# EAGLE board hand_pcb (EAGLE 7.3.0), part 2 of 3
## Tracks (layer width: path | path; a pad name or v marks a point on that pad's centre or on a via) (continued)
+5V1  (via drill 0.38, 0.39) (continued)
  pour Bottom (isolate 1.016, rank 2): 31.83,93.92 28.32,93.92 27.14,95.07 24.89,97.18 21.18,97.37 18.43,97.42 16.9,97.05 15.72,96.37 13.79,96.62 12.7,97.28 12.74,98.35 13.34,99.09 14.61,99.44 16.41,99.92 18.17,100.56 19.63,101.24 21.48,102.48 22.85,103.77 23.95,105.22 24.83,106.68 25.04,107.37 26.12,113.53 26.47,115.62 26.5,118.2 26.35,119.42 26.21,120.65 25.64,122.83 25.12,124.12 24.78,125.13 24.64,126.11 24.49,128.27 48.49,128.23 50.2,127.74 50.16,125.12 47.47,123.44 43.88,122.17 44.34,115.27 35.92,114.48 33.86,111.98 36.14,106.78 39.55,102.27 42.93,97.64 48.7,97.09 49.76,85.5 34.99,87.38
+5V2  (via drill 0.38, 0.39)
  Top 0.254: THMB2.15 111.18,51.43 110.49,52.12 110.49,55.24 109.67,56.07 107.34,56.07 v105.93,57.48 | PKYRNG2.15 119.56,21.16 119.25,20.85 112.03,20.85 111.76,21.12 111.76,25.86 112.52,26.62 C44.1 112.52,26.4 | 116.99,58.28 C47.1 116.6,59.2 v115.44,60.36 | 115.33,55.67 115.06,55.65 | INDMID2.15 81.54,21.43 80.2,22.77 80.48,26.57 82.16,28.14 82.16,29.65 82.58,30.07 85.8,30.07 87.55,28.32
  Top 0.381: 115.06,55.65 115.06,54.99 THMB2.10 | PKYRNG2.10 115.66,25.58 115.39,25.77 | C44.1 | INDMID2.10 86.06,25.43 86.26,25.45 | 87.52,27.5 87.73,27.72
  Top 0.762: 115.75,56.13 115.33,55.67 | 115.39,25.77 114.68,26.09 | 86.26,25.45 86.47,26.06
  Top 1.016: v133.32,55.52 134.73,55.52 C55.1
  Top 1.27: C42.2 C44.1 | C39.2 87.73,27.72 C41.1 | C47.1 117.39,58.28 C45.2 | 116.99,58.28 116.99,56.79 116.33,56.13 115.75,56.13 | 114.68,26.09 113.81,26.62 C44.1 | 86.47,26.06 87.35,27.09 87.52,27.5
  Top 1.524: C42.2 111.49,27.95 110.98,28.45 110.98,31.17 v111.01,31.19 | v89.98,31.08 88.35,31.08 87.55,29.59 87.55,28.32 87.55,27.89 87.73,27.72
  Top 1.905: 122.02,59.83 121.58,60.29 118.14,60.29 117.39,59.91 117.39,58.28
  Top 2.794: v122.03,58.78 122.02,58.55 122.02,59.83
  Bottom 0.254: v105.93,57.48 105.93,57.45 107.3,56.08 111.16,56.08 v115.44,60.36
  Bottom 1.016: v123.14,57.99 126.18,54.95 U$33.1 132.75,54.95 v133.32,55.52
  Bottom 1.524: 112.14,56.82 111.72,56.4 111.27,56.4 111.12,56.26 110.92,56.26 110.73,56.07 110.43,56.07 110.21,55.85 109.58,55.85 109.03,55.31 108.56,55.31
  Bottom 1.905: 113.53,57.2 113.14,56.82 112.14,56.82
  Bottom 2.794: v111.01,31.19 111.01,32.87 109.97,33.91 | 109.97,33.91 106.46,33.91 106.01,33.45 102.49,33.45 | 102.49,33.45 100.71,33.45 100.03,32.77 96.88,32.77 93.7,31.37 90.96,31.37 v89.98,31.08 | 109.97,33.91 110.01,33.95 | 103.34,40.88 103.34,50.98 | 103.34,50.98 103.34,51.13 | v122.03,58.78 113.51,58.76 113.53,58.75 113.53,57.2 | 108.56,55.31 104.23,50.98 103.34,50.98 | 103.85,40.37 102.49,39.01 102.49,33.45
  Bottom 3.81: U$28.3 106.01,28.65 106.01,33.45
  other vias: 104.85,31.24 107.2,30.19 89.26,30.04 107.24,32.13 111.05,32.58 91.35,30.73 90.98,32.28 88.38,31.34 120.68,59.65 121.31,57.77 123.19,59.35 122.07,60.12 118.66,59.88 117.16,59.92
  pour Top (isolate 0.406): 115.89,25.54 113.96,25.54 113.35,26.15 110.81,26.15 106.27,26.58 104.13,28.26 104.23,32.88 112.31,33.16 112.37,30.8 111.84,30.63 111.84,28.85 112.04,28.65 113.74,28.65 115.62,26.77 115.62,25.86 115.91,25.57
  pour Top (isolate 0.406): 85.98,24.97 85.98,26.64 86.35,27.01 86.35,30.57 88.07,32.03 91.52,32.92 92.11,32.5 92.48,30.91 91.87,30.12 90.61,29.1 88.75,28.96 88.75,26.39 87.85,25.49 86.6,25.49 86.08,24.97
  pour Top (isolate 0.406): 115.02,55.23 115.02,56.52 116,57.49 116,59.08 115.53,59.55 114.97,59.55 114.67,59.86 114.67,60.96 115.23,61.52 122.99,61.52 124.09,60.41 124.09,58.66 122.9,57.47 121.39,57.47 120.73,58.13 120.73,58.93 119.98,59.68 118.99,59.68 118.52,59.21 118.52,56.88 117.21,55.58 116.07,55.58 115.75,55.26 115.07,55.26 115.06,55.24
  pour Bottom (isolate 1.016, rank 2): 106.68,26.76 103.17,26.76 101.99,27.91 99.75,30.02 96.04,30.21 93.28,30.26 91.76,29.9 90.58,29.21 88.65,29.46 87.55,30.12 87.59,31.19 88.19,31.93 89.46,32.28 91.26,32.77 93.03,33.4 94.49,34.09 96.33,35.32 97.7,36.61 98.81,38.06 99.68,39.52 99.9,40.21 100.98,46.37 101.32,48.46 101.36,51.04 101.21,52.26 101.07,53.49 100.5,55.68 99.97,56.96 99.63,57.98 99.49,58.95 99.34,61.11 123.34,61.07 125.06,60.58 125.02,57.96 122.33,56.29 118.73,55.02 119.19,48.11 110.77,47.32 108.71,44.82 111,39.62 114.4,35.12 117.78,30.48 123.56,29.93 124.61,18.34 109.84,20.22
+5V3  (via drill 0.38, 0.39)
  Top 0.254: THMB3.15 110.41,82.05 111.1,81.36 111.1,78.23 111.92,77.41 114.25,77.41 v115.66,76 | PKYRNG3.15 102.03,112.32 102.34,112.62 109.56,112.62 109.83,112.36 109.83,107.62 109.07,106.86 C63.1 109.07,107.07 | 104.6,75.2 C66.1 104.99,74.27 v106.15,73.11 | 106.25,77.81 106.53,77.83 | INDMID3.15 140.05,112.05 141.39,110.71 141.11,106.91 139.43,105.33 139.43,103.82 139.01,103.4 135.79,103.4 134.04,105.16
  Top 0.381: 106.53,77.83 106.53,78.49 THMB3.10 | PKYRNG3.10 105.93,107.9 106.2,107.71 | C63.1 | INDMID3.10 135.53,108.05 135.33,108.03 | 134.07,105.98 133.86,105.76
  Top 0.762: 105.84,77.34 106.25,77.81 | 106.2,107.71 106.91,107.39 | 135.33,108.03 135.12,107.42
  Top 1.016: v88.27,77.95 86.86,77.95 C74.1
  Top 1.27: C61.2 C63.1 | C58.2 133.86,105.76 C60.1 | C66.1 104.2,75.2 C64.2 | 104.6,75.2 104.6,76.68 105.26,77.34 105.84,77.34 | 106.91,107.39 107.78,106.86 C63.1 | 135.12,107.42 134.24,106.39 134.07,105.98
  Top 1.524: C61.2 110.1,105.53 110.6,105.03 110.6,102.31 v110.58,102.29 | v131.61,102.4 133.24,102.4 134.04,103.89 134.04,105.16 134.04,105.58 133.86,105.76
  Top 1.905: 99.57,73.65 100.01,73.19 103.45,73.19 104.2,73.57 104.2,75.2
  Top 2.794: v99.56,74.7 99.57,74.93 99.57,73.65
  Bottom 0.254: v115.66,76 115.66,76.02 114.29,77.39 110.43,77.39 v106.15,73.11
  Bottom 1.016: v98.45,75.49 95.41,78.53 U$45.1 88.84,78.53 v88.27,77.95
  Bottom 1.524: 109.45,76.66 109.87,77.08 110.33,77.08 110.47,77.22 110.67,77.22 110.86,77.41 111.16,77.41 111.38,77.62 112.01,77.62 112.56,78.17 113.03,78.17
  Bottom 1.905: 108.06,76.28 108.44,76.66 109.45,76.66
  Bottom 2.794: v110.58,102.29 110.58,100.61 111.62,99.57 | 111.62,99.57 115.13,99.57 115.58,100.03 119.1,100.03 | 119.1,100.03 120.88,100.03 121.56,100.71 124.71,100.71 127.89,102.11 130.63,102.11 v131.61,102.4 | 111.62,99.57 111.58,99.53 | 118.25,92.6 118.25,82.5 | 118.25,82.5 118.25,82.35 | v99.56,74.7 108.08,74.71 108.06,74.73 108.06,76.28 | 113.03,78.17 117.36,82.5 118.25,82.5 | 117.74,93.1 119.1,94.46 119.1,100.03
  Bottom 3.81: U$40.3 115.58,104.83 115.58,100.03
  other vias: 116.74,102.23 114.39,103.29 132.33,103.44 114.35,101.35 110.54,100.9 130.24,102.74 130.61,101.19 133.21,102.13 100.91,73.83 100.28,75.7 98.4,74.13 99.52,73.36 102.93,73.6 104.43,73.56
  pour Top (isolate 0.406): 105.7,107.94 107.63,107.94 108.24,107.33 110.78,107.33 115.32,106.9 117.46,105.22 117.36,100.6 109.28,100.32 109.22,102.68 109.75,102.84 109.75,104.62 109.55,104.83 107.85,104.83 105.97,106.71 105.97,107.62 105.68,107.91
  pour Top (isolate 0.406): 135.61,108.51 135.61,106.83 135.24,106.46 135.24,102.91 133.52,101.45 130.07,100.56 129.48,100.98 129.11,102.57 129.72,103.35 130.98,104.38 132.84,104.52 132.84,107.09 133.74,107.99 134.99,107.99 135.51,108.51
  pour Top (isolate 0.406): 106.57,78.24 106.57,76.96 105.59,75.98 105.59,74.4 106.06,73.93 106.62,73.93 106.92,73.62 106.92,72.52 106.36,71.96 98.6,71.96 97.5,73.06 97.5,74.82 98.69,76.01 100.2,76.01 100.86,75.35 100.86,74.55 101.61,73.8 102.6,73.8 103.07,74.27 103.07,76.59 104.38,77.9 105.52,77.9 105.84,78.22 106.51,78.22 106.53,78.23
  pour Bottom (isolate 1.016, rank 2): 114.91,106.72 118.41,106.72 119.6,105.56 121.84,103.45 125.55,103.26 128.31,103.21 129.83,103.58 131.01,104.27 132.94,104.01 134.04,103.35 134,102.29 133.4,101.55 132.13,101.19 130.33,100.71 128.56,100.08 127.1,99.39 125.26,98.16 123.89,96.86 122.78,95.42 121.91,93.95 121.69,93.27 120.61,87.11 120.27,85.01 120.23,82.44 120.38,81.22 120.52,79.98 121.09,77.8 121.62,76.52 121.96,75.5 122.1,74.52 122.25,72.36 98.25,72.4 96.53,72.9 96.57,75.51 99.26,77.19 102.86,78.46 102.4,85.37 110.82,86.16 112.88,88.66 110.59,93.85 107.19,98.36 103.81,103 98.03,103.54 96.98,115.14 111.75,113.26
EN1
  Top 0.254: U$1.4 40.5,43.47 41.43,44.4 41.43,48.28 38.48,51.23 37.24,51.23 U$5.1
EN2
  Top 0.254: U$1.5 40.61,42.82 41.88,44.09 41.88,48.49 U$5.2
EN3
  Top 0.254: U$7.1 48.28,41.96 47.42,42.82 U$1.12
EN4
  Top 0.254: U$7.2 49.99,40.92 48.28,40.92 47.03,42.17 U$1.11
EN5  (via drill 0.38)
  Top 0.254: U$1.10 43.67,41.52 42.8,42.39 42.8,45.97 v43.08,46.25
  Bottom 0.254: v43.08,46.25 45.06,46.25 51.66,52.86 U$6.1
EN6  (via drill 0.38)
  Top 0.254: U$1.9 43.56,40.87 42.34,42.09 42.34,46.97 v42.62,47.24
  Bottom 0.254: v42.62,47.24 45.29,47.24 50.44,52.4 50.44,54.86 51.61,56.03 U$6.2
EN7
  Top 0.254: U$13.4 31.25,90.16 30.33,89.23 30.33,85.34 33.27,82.4 34.52,82.4 U$17.1
EN8
  Top 0.254: U$13.5 31.14,90.81 29.87,89.53 29.87,85.14 U$17.2
EN9  (via drill 0.38)
  Top 0.254: U$13.9 28.2,92.76 29.41,91.54 29.41,86.67 v29.13,86.39
  Bottom 0.254: v29.13,86.39 26.47,86.39 21.31,81.23 21.31,78.77 20.14,77.6 U$19.2
EN10
  Top 0.254: U$18.1 23.47,91.67 24.33,90.81 U$13.12
EN11
  Top 0.254: U$18.2 21.77,92.71 23.47,92.71 24.72,91.46 U$13.11
EN12  (via drill 0.38)
  Top 0.254: U$13.10 28.09,92.11 28.96,91.24 28.96,87.66 v28.68,87.38
  Bottom 0.254: v28.68,87.38 26.7,87.38 20.09,80.77 U$19.1
EN13
  Top 0.254: U$25.4 106.11,23 105.18,22.07 105.18,18.19 108.13,15.24 109.37,15.24 U$29.1
EN14
  Top 0.254: U$25.5 106,23.65 104.72,22.38 104.72,17.98 U$29.2
EN15  (via drill 0.38)
  Top 0.254: U$25.9 103.05,25.6 104.27,24.38 104.27,19.51 v103.99,19.23
  Bottom 0.254: v103.99,19.23 101.32,19.23 96.16,14.07 96.16,11.61 95,10.44 U$31.2
EN16
  Top 0.254: U$30.1 98.32,24.51 99.19,23.65 U$25.12
EN17
  Top 0.254: U$30.2 96.62,25.55 98.32,25.55 99.58,24.3 U$25.11
EN18  (via drill 0.38)
  Top 0.254: U$25.10 102.94,24.95 103.81,24.08 103.81,20.5 v103.53,20.22
  Bottom 0.254: v103.53,20.22 101.55,20.22 94.94,13.61 U$31.1
EN19
  Top 0.254: U$37.4 115.48,110.48 116.41,111.4 116.41,115.29 113.46,118.24 112.22,118.24 U$41.1
EN20
  Top 0.254: U$37.5 115.59,109.83 116.86,111.1 116.86,115.49 U$41.2
EN21  (via drill 0.38)
  Top 0.254: U$37.9 118.54,107.88 117.32,109.09 117.32,113.97 v117.6,114.25
  Bottom 0.254: v117.6,114.25 120.27,114.25 125.42,119.41 125.42,121.87 126.59,123.04 U$43.2
EN22
  Top 0.254: U$42.1 123.27,108.97 122.41,109.83 U$37.12
EN23
  Top 0.254: U$42.2 124.97,107.92 123.27,107.92 122.01,109.18 U$37.11
EN24  (via drill 0.38)
  Top 0.254: U$37.10 118.65,108.53 117.78,109.4 117.78,112.98 v118.06,113.26
  Bottom 0.254: v118.06,113.26 120.04,113.26 126.64,119.86 U$43.1
GND  (via drill 0.3, 0.38, 0.39, 1.27)
  Top 0.254: THUMB_A.6 40.18,17.32 40.18,17.78 v40.79,18.39 | v41.83,30.5 41.56,29.7 THUMB_B.6 | BOOTLOADER.2 9.55,20.18 10.46,19.27 10.46,18.39 v10.71,18.15 12.56,18.96 C15.2 | 9.55,22.81 9.88,23.14 BOOTLOADER.PPAD | C15.2 13.42,19.61 | 29.64,41.55 PKYRNG.11 29.67,41.55 30.2,41.53 | PKYRNG.PPAD 27.73,41.22 28.07,41.55 26.94,41.55 v26.87,41.72 | HAND_MICRO.4 24.13,31.62 C14.2 24.38,32.56 v24.38,33.58 | HAND_MICRO.47 25.13,15.78 C16.2 25.4,15.22 v26.06,14.26 | INDMID.PPAD 60.88,44.73 v60.38,45.23 | HAND_MICRO.31 14.58,19.97 14.19,19.57 C15.2 | C15.2 | v47.16,38.08 47.13,38.1 44.32,38.1 41.55,40.87 U$1.8 37.74,40.87 37.06,41.55 C19.2
  Top 0.381: C3.2 61.2,38.91 | C2.2 61.79,37.4 61.37,37.82 C3.2 | PKYRNG.11 31.52,41.54 v32.79,44.01 32.35,41.9 33.45,41.53 C6.2 C5.2 | THMB.PPAD 31.88,14.82 v31.38,15.21 | v33.16,5.64 33.16,6.65 C8.2 33.03,6.87 C9.2 32.2,8.69 THMB.11 | INDMID.11 61.2,41.08 v61.73,40.55 61.35,40.17 C3.2 | INDEX.6 54.42,51.92 v54.41,51.93 | v41.17,52.41 41.66,50.95 42.4,50.86 MIDDLE.6 | RING.6 v25.52,49.76 v25.51,49.76 | v12.45,43.67 12.53,43.76 PINKY.6 13.46,43.72 13.46,41.2 13.42,41.16 13.42,40.4 16.03,37.79 U$3.1 | v5.94,38.28 6.19,38.03 USB.5 | C13.2 12.47,28.77 12.47,29.65 11.19,30.94 10.06,30.94 | 10.06,30.94 v12.12,30.71 | GND.P$1 10.06,30.94 | BOOTLOADER.PPAD 9.28,23.72 v9.28,24.31 v10.46,24.31 v10.46,23.13 v9.27,23.13
  Top 1.016: C17.2 12.08,8.7 v12.5,9.25 11.04,8.7 C18.2
  Route15 0.254: v41.83,30.5 42.34,30.76 44.76,30.76 | v26.87,40.72 26.89,40.73 27.84,40.73 27.85,40.74 27.85,40.84 | v24.38,33.58 25.45,32.51 v29.81,32.51 | v10.71,18.15 10.46,18.39 v10.46,23.13 | U$7.G 50.6,47.24 52.02,47.24 55.27,43.99 55.37,43.99
  Route15 0.381: v32.79,44.01 29.81,39.83 29.81,38.47 | v33.16,5.64 31.38,7.24 v31.38,15.21 | v61.73,40.55 61.73,42.09 60.54,43.28 60.54,45.06 v60.38,45.23 | v54.41,51.93 42.24,51.93 v41.17,52.41 40.07,49.76 v25.51,49.76 | v25.51,49.76 19.43,43.67 v12.45,43.67 12.45,42.99 9.51,39.8 v5.94,38.28 6.48,37.24 7.79,34.59 8.55,33.05 v12.12,30.71 | v25.51,49.76 25.54,49.73 25.54,45.5 26.87,44.17 v26.87,41.72 | v40.79,18.39 41.11,18.71 43.16,18.71
  Route15 0.762: v9.27,23.13 9.3,23.14 10.11,23.95 10.11,24.3 6.69,27.71 6.69,33.49 7.79,34.59
  Route15 1.524: v26.87,41.72 26.86,41.59 27.36,41.1
  Route15 2.794: 44.76,32.11 44.76,30.76 44.76,25.01 43.16,23.41 43.16,18.71 43.16,14.78 43.07,14.87 33.47,14.87 33.12,15.21 v31.38,15.21 | 44.76,32.11 50.87,38.22 53.3,40.4 53.3,41.92 55.37,43.99 55.75,44.37 60.54,44.37 INDMID.PPAD 60.88,44.73 v60.38,45.23 | 44.76,32.11 44.08,32.78 40.4,32.47 40.13,32.21 37.6,32.23 36.94,31.57 33.19,31.57 32.24,32.51 v29.81,32.51 29.81,38.47 29.81,38.65 27.36,41.1
  Route15 3.81: v48.35,38.7 50.87,38.66 50.87,38.22
  Bottom 0.254: v26.06,14.26 27.75,14.41 R5.1 | 35.69,19.79 39.4,19.79 v40.79,18.39 | R15.2 32.89,23.67 33.25,23.42 35.2,23.42 35.72,23.94 R14.2 35.72,26.14 R16.2 40.09,30.5 v41.83,30.5
  Bottom 1.016: U$9.2 U$9.TAB 9.09,11.79 10.08,12.78 10.03,17.48 v10.71,18.15
  Bottom 1.27: v31.38,15.21 31.77,13.79 32.26,13.31 | U$10.G 38.12,45.24 40.08,43.28 43.92,43.28 47.52,39.67
  Bottom 1.524: R9.1 R8.1 28.78,33.54 v29.81,32.51 | R7.1 61.61,43.28 | 61.61,43.28 R6.1 | R5.1 28.85,13.31 32.26,13.31 R4.1 34.95,13.34 | v60.38,45.23 60.35,44.54 61.61,43.28
  Bottom 3.81: U$2.1 43.87,42.76 43.87,42.72 v48.35,38.7
  other vias: 49.7,38.68 48.69,37.49 48.97,40.01 47.41,39.7 60.38,44.21 61.38,44.21 61.38,45.22 32.38,14.21 32.38,15.21 31.38,14.21 27.88,41.72 27.88,40.72 29.13,33.4 29.18,36.5 10.03,15.54 10.03,13.21 65.53,48.44 29.62,35.05 7.04,27.74 42.85,7.16
  pour Route15 (isolate 0.508): 4.58,49.38 6.54,8.14 9.13,5.23 47.61,5.17 47.04,8.65 45.47,13.96 45.59,18.88 46.72,26.29 49.31,30.28 52.29,32.42 56.39,33.57 62.97,35.59 66.56,36.6 67.83,62.98 54.05,63.61 53.73,58.36 23.22,56.78 23.28,50.27
  pour Bottom (isolate 1.016, rank 3): 36.8,49.25 36.8,46.84 37.49,46.15 37.49,41.86 38.61,40.74 43.1,40.74 46.15,37.69 46.15,37.67 47.88,35.94 48.79,35.94 50.6,37.74 50.6,39.78 50.14,40.23 50.14,46.79 47.42,49.5 38.71,49.5
GND1  (via drill 0.3, 0.38, 0.39, 1.27)
  Top 0.254: THUMB_A1.6 31.57,116.31 31.57,115.85 v30.96,115.24 | v29.92,103.12 30.2,103.93 THUMB_B1.6 | BOOTLOADER1.2 62.2,113.45 61.29,114.36 61.29,115.24 v61.05,115.48 59.2,114.67 C34.2 | 62.2,110.82 61.88,110.49 BOOTLOADER1.PPAD | C34.2 58.33,114.02 | 42.12,92.08 PKYRNG1.11 42.09,92.08 41.55,92.1 | PKYRNG1.PPAD 44.03,92.41 43.69,92.08 44.82,92.08 v44.88,91.91 | HAND_MICRO1.4 47.63,102.01 C33.2 47.37,101.07 v47.37,100.05 | HAND_MICRO1.47 46.63,117.85 C35.2 46.35,118.4 v45.7,119.37 | INDMID1.PPAD 10.88,88.89 v11.38,88.41 | HAND_MICRO1.31 57.17,113.66 57.57,114.06 C34.2 | C34.2 | v24.6,95.56 24.62,95.53 27.43,95.53 30.2,92.76 U$13.8 34.01,92.76 34.7,92.08 C38.2
  Top 0.381: C22.2 10.55,94.72 | C21.2 9.97,96.23 10.39,95.81 10.39,94.89 C22.2 | PKYRNG1.11 40.23,92.09 v38.96,89.62 39.41,91.73 38.3,92.1 C25.2 C24.2 | THMB1.PPAD 39.88,118.81 v40.37,118.42 | v38.59,127.99 38.59,126.98 C27.2 38.72,126.76 C28.2 39.55,124.94 THMB1.11 | INDMID1.11 10.55,92.55 v10.02,93.08 10.4,93.46 C22.2 | INDEX1.6 17.33,81.71 v17.35,81.7 | v30.58,81.22 30.1,82.68 29.35,82.77 MIDDLE1.6 | RING1.6 v46.24,83.87 | v59.31,89.95 59.22,89.87 PINKY1.6 58.29,89.91 58.29,92.43 58.33,92.47 58.33,93.23 55.73,95.83 U$14.1 | v65.81,95.35 65.57,95.59 USB1.5 | C32.2 59.28,104.86 59.28,103.97 60.57,102.69 61.7,102.69 | 61.7,102.69 v59.64,102.92 | GND1.P$1 61.7,102.69 | BOOTLOADER1.PPAD 62.47,109.91 v62.47,109.32 v61.29,109.32 v61.29,110.5 v62.48,110.5
  Top 1.016: C36.2 59.68,124.93 v59.26,124.38 60.72,124.93 C37.2
  Route15 0.254: v29.92,103.12 29.41,102.87 27,102.87 | v44.88,92.91 v44.87,92.9 43.92,92.9 43.9,92.89 43.9,92.79 | v47.37,100.05 46.3,101.12 v41.95,101.12 | v61.05,115.48 61.29,115.24 v61.29,110.5 | U$18.G 21.16,86.39 19.74,86.39 16.48,89.64 16.38,89.64
  Route15 0.381: v38.96,89.62 41.95,93.8 41.95,95.16 | v38.59,127.99 40.37,126.39 v40.37,118.42 | v10.02,93.08 10.02,91.54 11.21,90.35 11.21,88.57 v11.38,88.41 | v17.35,81.7 29.52,81.7 v30.58,81.22 31.69,83.87 v46.24,83.87 | v46.24,83.87 52.32,89.95 v59.31,89.95 59.31,90.64 62.24,93.83 v65.81,95.35 65.28,96.39 63.97,99.04 63.21,100.58 v59.64,102.92 | v46.24,83.87 46.22,83.9 46.22,88.12 44.88,89.46 v44.88,91.91 | v30.96,115.24 30.64,114.92 28.6,114.92
  Route15 0.762: v62.48,110.5 62.46,110.49 61.65,109.68 61.65,109.33 65.06,105.92 65.06,100.14 63.97,99.04
  Route15 1.524: v44.88,91.91 44.9,92.04 44.4,92.53
  Route15 2.794: 27,101.52 27,102.87 27,108.62 28.6,110.22 28.6,114.92 28.6,118.85 28.69,118.76 38.29,118.76 38.63,118.42 v40.37,118.42 | 27,101.52 20.89,95.41 18.45,93.23 18.45,91.71 16.38,89.64 16,89.26 11.22,89.26 INDMID1.PPAD 10.88,88.89 v11.38,88.41 | 27,101.52 27.67,100.85 31.36,101.16 31.62,101.42 34.15,101.4 34.81,102.06 38.57,102.06 39.51,101.12 v41.95,101.12 41.95,95.16 41.95,94.98 44.4,92.53
  Route15 3.81: v23.41,94.93 20.89,94.96 20.89,95.41
  Bottom 0.254: v45.7,119.37 44.01,119.22 R21.1 | 36.07,113.84 32.36,113.84 v30.96,115.24 | R31.2 38.86,109.96 38.51,110.21 36.55,110.21 36.03,109.69 R30.2 36.03,107.49 R32.2 31.66,103.12 v29.92,103.12
  Bottom 1.016: U$21.2 U$21.TAB 62.66,121.84 61.67,120.85 61.72,116.15 v61.05,115.48
  Bottom 1.27: v40.37,118.42 39.98,119.84 39.5,120.32 | U$22.G 33.63,88.39 31.67,90.35 27.84,90.35 24.23,93.95
  Bottom 1.524: R25.1 R24.1 42.98,100.09 v41.95,101.12 | R23.1 10.15,90.35 | 10.15,90.35 R22.1 | R21.1 42.9,120.32 39.5,120.32 R20.1 36.8,120.29 | v11.38,88.41 11.4,89.09 10.15,90.35
  Bottom 3.81: U$16.1 27.89,90.87 27.89,90.91 v23.41,94.93
  other vias: 22.06,94.95 23.06,96.14 22.78,93.62 24.35,93.93 11.38,89.42 10.38,89.42 10.38,88.4 39.37,119.42 39.37,118.41 40.37,119.42 43.88,91.91 43.88,92.91 42.62,100.23 42.57,97.13 61.72,118.08 61.72,120.42 6.22,85.19 42.14,98.58 64.72,105.89 28.91,126.47
  pour Route15 (isolate 0.508): 67.17,84.25 65.21,125.49 62.62,128.4 24.14,128.46 24.71,124.98 26.29,119.67 26.16,114.74 25.03,107.34 22.44,103.35 19.47,101.21 15.37,100.06 8.79,98.04 5.19,97.03 3.92,70.65 17.7,70.02 18.02,75.27 48.54,76.85 48.48,83.36
  pour Bottom (isolate 1.016, rank 3): 34.95,84.38 34.95,86.79 34.26,87.48 34.26,91.77 33.15,92.89 28.65,92.89 25.6,95.94 25.6,95.96 23.88,97.69 22.96,97.69 21.16,95.89 21.16,93.85 21.62,93.4 21.62,86.84 24.33,84.12 33.05,84.12
GND2  (via drill 0.3, 0.38, 0.39, 1.27)
  Top 0.254: THUMB_A2.6 106.43,49.15 106.43,48.69 v105.82,48.08 | v104.78,35.97 105.05,36.78 THUMB_B2.6 | BOOTLOADER2.2 137.06,46.29 136.14,47.21 136.14,48.08 v135.9,48.32 134.05,47.51 C53.2 | 137.06,43.66 136.73,43.34 BOOTLOADER2.PPAD | C53.2 133.19,46.86 | 116.97,24.92 PKYRNG2.11 116.94,24.92 116.41,24.94 | PKYRNG2.PPAD 118.88,25.25 118.54,24.92 119.67,24.92 v119.74,24.75 | HAND_MICRO2.4 122.48,34.85 C52.2 122.22,33.91 v122.22,32.89 | HAND_MICRO2.47 121.48,50.69 C54.2 121.21,51.25 v120.55,52.21 | INDMID2.PPAD 85.73,21.74 v86.23,21.25 | HAND_MICRO2.31 132.03,46.51 132.42,46.9 C53.2 | C53.2 | v99.45,28.4 99.48,28.37 102.29,28.37 105.06,25.6 U$25.8 108.87,25.6 109.55,24.92 C57.2
  Top 0.381: C41.2 85.41,27.57 | C40.2 84.82,29.07 85.24,28.65 C41.2 | PKYRNG2.11 115.09,24.93 v113.82,22.47 114.26,24.57 113.16,24.94 C44.2 C43.2 | THMB2.PPAD 114.73,51.65 v115.23,51.26 | v113.45,60.83 113.45,59.82 C46.2 113.57,59.6 C47.2 114.41,57.78 THMB2.11 | INDMID2.11 85.41,25.39 v84.87,25.92 85.25,26.3 C41.2 | INDEX2.6 92.19,14.55 v92.2,14.54 | v105.44,14.06 104.95,15.52 104.21,15.61 MIDDLE2.6 | RING2.6 v121.09,16.71 | v134.16,22.8 134.08,22.71 PINKY2.6 133.15,22.75 133.15,25.27 133.19,25.31 133.19,26.07 130.58,28.68 U$26.1 | v140.66,28.19 140.42,28.44 USB2.5 | C51.2 134.14,37.7 134.14,36.82 135.42,35.53 136.55,35.53 | 136.55,35.53 v134.49,35.76 | GND2.P$1 136.55,35.53 | BOOTLOADER2.PPAD 137.32,42.76 v137.32,42.16 v136.14,42.16 v136.14,43.34 v137.34,43.34
  Top 1.016: C55.2 134.53,57.77 v134.11,57.23 135.57,57.77 C56.2
  Route15 0.254: v104.78,35.97 104.27,35.71 101.85,35.71 | v119.74,25.76 119.72,25.74 118.77,25.74 118.76,25.73 118.76,25.63 | v122.22,32.89 121.16,33.96 v116.8,33.96 | v135.9,48.32 136.14,48.08 v136.14,43.34 | U$30.G 96.01,19.23 94.59,19.23 91.34,22.48 91.24,22.48
  Route15 0.381: v113.82,22.47 116.8,26.64 116.8,28 | v113.45,60.83 115.23,59.23 v115.23,51.26 | v84.87,25.92 84.87,24.38 86.07,23.19 86.07,21.41 v86.23,21.25 | v92.2,14.54 104.37,14.54 v105.44,14.06 106.54,16.71 v121.09,16.71 | v121.09,16.71 127.18,22.8 v134.16,22.8 134.16,23.48 137.1,26.67 v140.66,28.19 140.13,29.23 138.82,31.89 138.06,33.43 v134.49,35.76 | v121.09,16.71 121.07,16.74 121.07,20.97 119.74,22.3 v119.74,24.75 | v105.82,48.08 105.5,47.77 103.45,47.77
  Route15 0.762: v137.34,43.34 137.31,43.33 136.5,42.52 136.5,42.18 139.92,38.76 139.92,32.98 138.82,31.89
  Route15 1.524: v119.74,24.75 119.75,24.88 119.25,25.38
  Route15 2.794: 101.85,34.37 101.85,35.71 101.85,41.47 103.45,43.07 103.45,47.77 103.45,51.69 103.54,51.6 113.14,51.6 113.49,51.26 v115.23,51.26 | 101.85,34.37 95.74,28.25 93.31,26.07 93.31,24.55 91.24,22.48 90.86,22.1 86.07,22.1 INDMID2.PPAD 85.73,21.74 v86.23,21.25 | 101.85,34.37 102.53,33.69 106.21,34 106.48,34.27 109,34.24 109.67,34.9 113.42,34.9 114.36,33.96 v116.8,33.96 116.8,28 116.8,27.83 119.25,25.38
  Route15 3.81: v98.26,27.77 95.74,27.81 95.74,28.25
  Bottom 0.254: v120.55,52.21 118.86,52.06 R37.1 | 110.92,46.69 107.21,46.69 v105.82,48.08 | R47.2 113.72,42.8 113.36,43.05 111.4,43.05 110.89,42.53 R46.2 110.89,40.34 R48.2 106.52,35.97 v104.78,35.97
  Bottom 1.016: U$33.2 U$33.TAB 137.51,54.69 136.53,53.7 136.57,48.99 v135.9,48.32
  Bottom 1.27: v115.23,51.26 114.83,52.68 114.35,53.16 | U$34.G 108.48,21.23 106.53,23.19 102.69,23.19 99.08,26.8
  Bottom 1.524: R41.1 R40.1 117.83,32.93 v116.8,33.96 | R39.1 85,23.19 | 85,23.19 R38.1 | R37.1 117.75,53.16 114.35,53.16 R36.1 111.66,53.14 | v86.23,21.25 86.26,21.93 85,23.19
  Bottom 3.81: U$28.1 102.74,23.71 102.74,23.75 v98.26,27.77
  other vias: 96.91,27.79 97.92,28.98 97.64,26.47 99.2,26.77 86.23,22.26 85.23,22.26 85.23,21.25 114.22,52.26 114.22,51.26 115.23,52.26 118.73,24.75 118.73,25.76 117.47,33.07 117.42,29.97 136.58,50.93 136.58,53.26 81.08,18.03 116.99,31.42 139.57,38.73 103.76,59.31
  pour Route15 (isolate 0.508): 142.02,17.09 140.07,58.33 137.48,61.24 99,61.3 99.57,57.82 101.14,52.51 101.02,47.59 99.89,40.18 97.29,36.2 94.32,34.05 90.22,32.91 83.64,30.89 80.05,29.87 78.78,3.49 92.56,2.86 92.88,8.12 123.39,9.69 123.33,16.21
  pour Bottom (isolate 1.016, rank 3): 109.8,17.22 109.8,19.63 109.12,20.32 109.12,24.61 108,25.73 103.5,25.73 100.46,28.78 100.46,28.8 98.73,30.53 97.82,30.53 96.01,28.73 96.01,26.7 96.47,26.24 96.47,19.68 99.19,16.97 107.9,16.97
GND3  (via drill 0.3, 0.38, 0.39, 1.27)
  Top 0.254: THUMB_A3.6 115.16,84.33 115.16,84.78 v115.77,85.39 | v116.81,97.51 116.54,96.7 THUMB_B3.6 | BOOTLOADER3.2 84.53,87.18 85.45,86.27 85.45,85.39 v85.69,85.15 87.54,85.97 C72.2 | 84.53,89.81 84.86,90.14 BOOTLOADER3.PPAD | C72.2 88.4,86.61 | PKYRNG3.11 104.65,108.56 105.18,108.53 | PKYRNG3.PPAD 102.71,108.22 103.05,108.56 101.92,108.56 v101.85,108.72 | HAND_MICRO3.4 99.11,98.62 C71.2 99.36,99.57 v99.36,100.58 | HAND_MICRO3.47 100.11,82.78 C73.2 100.38,82.23 v101.04,81.27 | INDMID3.PPAD 135.86,111.74 v135.36,112.23 | HAND_MICRO3.31 89.56,86.97 89.17,86.58 C72.2 | C72.2 | v122.14,105.08 122.11,105.11 119.3,105.11 116.53,107.88 U$37.8 112.72,107.88 112.04,108.56 C76.2
  Top 0.381: C60.2 136.18,105.91 | C59.2 136.77,104.41 136.35,104.83 136.35,105.75 C60.2 | PKYRNG3.11 106.5,108.55 v107.77,111.01 107.33,108.9 108.43,108.53 C63.2 C62.2 | THMB3.PPAD 106.86,81.83 v106.36,82.22 | v108.14,72.64 108.14,73.65 C65.2 108.02,73.87 C66.2 107.18,75.7 THMB3.11 | INDMID3.11 136.18,108.09 v136.72,107.56 136.34,107.18 C60.2 | INDEX3.6 129.4,118.92 v129.39,118.94 | v116.15,119.42 116.64,117.96 117.38,117.87 MIDDLE3.6 | RING3.6 v100.5,116.77 v100.5,116.76 | v87.43,110.68 87.51,110.77 PINKY3.6 88.44,110.73 88.44,108.2 88.41,108.17 88.41,107.4 91.01,104.8 U$38.1 | v80.92,105.28 81.17,105.04 USB3.5 | C70.2 87.45,95.78 87.45,96.66 86.17,97.94 85.04,97.94 | 85.04,97.94 v87.1,97.71 | GND3.P$1 85.04,97.94 | BOOTLOADER3.PPAD 84.26,90.72 v84.26,91.31 v85.45,91.31 v85.45,90.13 v84.25,90.13
  Top 1.016: C74.2 87.06,75.71 v87.48,76.25 86.02,75.7 C75.2
  Route15 0.254: v116.81,97.51 117.32,97.77 119.74,97.77 | v101.85,107.72 101.87,107.73 102.82,107.73 102.83,107.75 102.83,107.85 | v99.36,100.58 100.43,99.52 v104.79,99.52 | v85.69,85.15 85.45,85.39 v85.45,90.13 | U$42.G 125.58,114.25 127,114.25 130.25,111 130.35,111
  Route15 0.381: v107.77,111.01 104.79,106.83 104.79,105.47 | v108.14,72.64 106.36,74.24 v106.36,82.22 | v136.72,107.56 136.72,109.09 135.52,110.29 135.52,112.06 v135.36,112.23 | v129.39,118.94 117.22,118.94 v116.15,119.42 115.05,116.76 v100.5,116.76 | v100.5,116.76 94.41,110.68 v87.43,110.68 87.43,110 84.49,106.81 v80.92,105.28 81.46,104.24 82.77,101.59 83.53,100.05 v87.1,97.71 | v100.5,116.76 100.52,116.74 100.52,112.51 101.85,111.18 v101.85,108.72 | v115.77,85.39 116.09,85.71 118.14,85.71
  Route15 0.762: v84.25,90.13 84.28,90.14 85.09,90.96 85.09,91.3 81.67,94.72 81.67,100.5 82.77,101.59
  Route15 1.524: v101.85,108.72 101.84,108.6 102.34,108.1
  Route15 2.794: 119.74,99.11 119.74,97.77 119.74,92.01 118.14,90.41 118.14,85.71 118.14,81.79 118.05,81.88 108.44,81.88 108.1,82.22 v106.36,82.22 | 119.74,99.11 125.85,105.23 128.28,107.4 128.28,108.93 130.35,111 130.73,111.38 135.52,111.38 INDMID3.PPAD 135.86,111.74 v135.36,112.23 | 119.74,99.11 119.06,99.78 115.38,99.48 115.11,99.21 112.58,99.24 111.92,98.58 108.17,98.58 107.23,99.52 v104.79,99.52 104.79,105.47 104.79,105.65 102.34,108.1
  Route15 3.81: v123.33,105.7 125.85,105.67 125.85,105.23
  Bottom 0.254: v101.04,81.27 102.73,81.42 R53.1 | 110.67,86.79 114.38,86.79 v115.77,85.39 | R63.2 107.87,90.68 108.23,90.42 110.19,90.42 110.7,90.94 R62.2 110.7,93.14 R64.2 115.07,97.51 v116.81,97.51
  Bottom 1.016: U$45.2 U$45.TAB 84.08,78.79 85.06,79.78 85.02,84.48 v85.69,85.15
  Bottom 1.27: v106.36,82.22 106.76,80.8 107.24,80.31 | U$46.G 113.11,112.24 115.06,110.29 118.9,110.29 122.5,106.68
  Bottom 1.524: R57.1 R56.1 103.76,100.55 v104.79,99.52 | R55.1 136.59,110.29 | 136.59,110.29 R54.1 | R53.1 103.83,80.31 107.24,80.31 R52.1 109.93,80.34 | v135.36,112.23 135.33,111.54 136.59,110.29
  Bottom 3.81: U$40.1 118.85,109.77 118.85,109.73 v123.33,105.7
  other vias: 124.68,105.69 123.67,104.5 123.95,107.01 122.39,106.71 135.36,111.21 136.36,111.21 136.36,112.23 107.37,81.22 107.37,82.22 106.36,81.22 102.86,108.72 102.86,107.72 104.11,100.41 104.17,103.5 85.01,82.55 85.01,80.21 140.51,115.44 104.6,102.06 82.02,94.74 117.83,74.17
  pour Route15 (isolate 0.508): 79.57,116.38 81.52,75.15 84.11,72.24 122.59,72.17 122.02,75.65 120.45,80.96 120.57,85.89 121.7,93.29 124.29,97.28 127.27,99.43 131.37,100.57 137.95,102.59 141.54,103.61 142.81,129.98 129.03,130.62 128.71,125.36 98.2,123.79 98.26,117.27
  pour Bottom (isolate 1.016, rank 3): 111.79,116.26 111.79,113.84 112.47,113.16 112.47,108.86 113.59,107.75 118.08,107.75 121.13,104.7 121.13,104.67 122.86,102.95 123.77,102.95 125.58,104.75 125.58,106.78 125.12,107.24 125.12,113.79 122.4,116.51 113.69,116.51
IDX1
  Top 0.254: 63.75,46.02 INDMID.16
  Top 0.635: 63.75,46.02 64.06,46.79 64.01,48.34 62.81,48.92 62.81,50.19 61.38,51.59 INDEX.1
IDX2
  Top 0.254: INDMID.2 61.21,46.99
  Top 0.381: 61.21,46.99 61.21,47.83 61.47,48.67
  Top 0.635: 61.47,48.67 61.47,49.17 60.66,49.94 60.18,50.32 INDEX.2
IDX3
  Top 0.254: 8,87.61 INDMID1.16
  Top 0.635: 8,87.61 7.7,86.84 7.75,85.29 8.94,84.71 8.94,83.44 10.38,82.04 INDEX1.1
IDX4
  Top 0.254: INDMID1.2
  Top 0.381: INDMID1.2 10.54,85.8 10.29,84.96
  Top 0.635: 10.29,84.96 10.29,84.45 11.1,83.69 11.58,83.31 INDEX1.2
IDX5
  Top 0.254: 82.86,20.45 INDMID2.16
  Top 0.635: 82.86,20.45 82.55,19.68 82.6,18.14 83.8,17.55 83.8,16.28 85.23,14.88 INDEX2.1
IDX6
  Top 0.254: INDMID2.2 85.39,19.48
  Top 0.381: 85.39,19.48 85.39,18.64 85.14,17.8
  Top 0.635: 85.14,17.8 85.14,17.3 85.95,16.54 86.43,16.15 INDEX2.2
IDX7
  Top 0.254: 138.74,113.03 INDMID3.16
  Top 0.635: 138.74,113.03 139.04,113.79 138.99,115.34 137.79,115.93 137.79,117.2 136.36,118.59 INDEX3.1
IDX8
  Top 0.254: INDMID3.2 136.19,114
  Top 0.381: 136.19,114 136.19,114.83 136.45,115.67
  Top 0.635: 136.45,115.67 136.45,116.18 135.64,116.94 135.16,117.32 INDEX3.2
IDXENC1  (via drill 0.38)
  Top 0.254: INDEX.5 v56.5,50.44 | HAND_MICRO.58 29.99,23.97 v30.71,24.69
  Route2 0.254: v30.71,24.69 42.04,24.69 54.48,37.13 54.48,46.25 57.15,48.92 57.15,49.8 v56.5,50.44
IDXENC2  (via drill 0.38)
  Top 0.254: INDEX.4 57.78,51.07 v57.78,50.39 | HAND_MICRO.57 26.06,23.47 v25.27,22.68
  Route2 0.254: v25.27,22.68 26.04,23.44 30.63,23.44 31.39,24.21 42.29,24.21 54.94,36.85 54.94,45.95 57.61,48.62 v57.78,50.39
IDXENC3  (via drill 0.38)
  Top 0.254: INDEX1.4 13.98,82.56 v13.97,83.24 | HAND_MICRO1.57 45.7,110.16 v46.48,110.95
  Route2 0.254: v46.48,110.95 45.72,110.19 41.12,110.19 40.36,109.42 29.46,109.42 16.82,96.77 16.82,87.68 14.15,85.01 v13.97,83.24
IDXENC4  (via drill 0.38)
  Top 0.254: INDEX1.5 v15.25,83.19 | HAND_MICRO1.58 41.77,109.66 v41.05,108.94
  Route2 0.254: v41.05,108.94 29.72,108.94 17.27,96.5 17.27,87.38 14.61,84.71 14.61,83.83 v15.25,83.19
IDXENC5  (via drill 0.38)
  Top 0.254: INDEX2.4 88.83,15.4 v88.82,16.08 | HAND_MICRO2.57 120.55,43.01 v121.34,43.79
  Route2 0.254: v121.34,43.79 120.57,43.03 115.98,43.03 115.21,42.27 104.32,42.27 91.67,29.62 91.67,20.52 89,17.86 v88.82,16.08
IDXENC6  (via drill 0.38)
  Top 0.254: INDEX2.5 v90.11,16.03 | HAND_MICRO2.58 116.62,42.51 v115.9,41.78
  Route2 0.254: v115.9,41.78 104.57,41.78 92.13,29.34 92.13,20.22 89.46,17.55 89.46,16.67 v90.11,16.03
IDXENC7  (via drill 0.38)
  Top 0.254: INDEX3.4 132.76,118.08 v132.77,117.4 | HAND_MICRO3.57 101.04,90.47 v100.25,89.69
  Route2 0.254: v100.25,89.69 101.02,90.45 105.61,90.45 106.38,91.21 117.27,91.21 129.92,103.86 129.92,112.95 132.59,115.62 v132.77,117.4
IDXENC8  (via drill 0.38)
  Top 0.254: INDEX3.5 v131.48,117.45 | HAND_MICRO3.58 104.97,90.97 v105.69,91.69
  Route2 0.254: v105.69,91.69 117.02,91.69 129.46,104.14 129.46,113.26 132.13,115.93 132.13,116.8 v131.48,117.45
IDXISEN  (via drill 0.38)
  Top 0.381: INDMID.1 62.08,47.57
  Top 0.635: 62.08,47.57 v62.74,47.47
  Bottom 0.635: v62.74,47.47 63.93,46.28 R6.2
IDXISEN1  (via drill 0.38)
  Top 0.381: INDMID1.1 9.68,86.06
  Top 0.635: 9.68,86.06 v9.02,86.16
  Bottom 0.635: v9.02,86.16 7.82,87.35 R22.2
IDXISEN2  (via drill 0.38)
  Top 0.381: INDMID2.1 84.53,18.9
  Top 0.635: 84.53,18.9 v83.87,19
  Bottom 0.635: v83.87,19 82.68,20.19 R38.2
IDXISEN3  (via drill 0.38)
  Top 0.381: INDMID3.1 137.06,114.58
  Top 0.635: 137.06,114.58 v137.72,114.48
  Bottom 0.635: v137.72,114.48 138.91,113.28 R54.2
IDXPWM1  (via drill 0.38)
  Top 0.254: INDMID.14 64.65,44.39 65.76,43.28 65.44,40.64 v64.87,40.02 | HAND_MICRO.61 28.97,25.47 34.8,31.29 48.49,31.29 55.63,38.43 55.63,40.36 v55.85,40.36
  Route2 0.254: 65.02,40.16 v64.87,40.02 63.45,38.58 57.33,38.58 v55.85,40.36
IDXPWM2  (via drill 0.38)
  Top 0.254: INDMID.13 63.15,42.77 v64.59,41.33 | HAND_MICRO.62 27.67,25.96 28.73,25.96 34.54,31.77 48.28,31.77 55.14,38.63 55.14,40.82 v55.73,41.4
  Route2 0.254: v55.73,41.4 64.54,41.38 v64.59,41.33
IDXPWM3  (via drill 0.38)
  Top 0.254: INDMID1.13 8.6,90.86 v7.16,92.3 | HAND_MICRO1.62 44.08,107.67 43.03,107.67 37.21,101.85 23.47,101.85 16.61,95 16.61,92.81 v16.03,92.23
  Route2 0.254: v16.03,92.23 7.21,92.25 v7.16,92.3
IDXPWM4  (via drill 0.38)
  Top 0.254: INDMID1.14 7.1,89.24 5.99,90.35 6.31,92.99 v6.88,93.61 | HAND_MICRO1.61 42.78,108.16 36.96,102.34 23.27,102.34 16.13,95.2 16.13,93.27 v15.9,93.27
  Route2 0.254: 6.73,93.47 v6.88,93.61 8.31,95.05 14.43,95.05 v15.9,93.27
IDXPWM5  (via drill 0.38)
  Top 0.254: INDMID2.13 83.46,23.71 v82.02,25.15 | HAND_MICRO2.62 118.94,40.51 117.88,40.51 112.06,34.7 98.32,34.7 91.47,27.84 91.47,25.65 v90.88,25.07
  Route2 0.254: v90.88,25.07 82.07,25.09 v82.02,25.15
IDXPWM6  (via drill 0.38)
  Top 0.254: INDMID2.14 81.96,22.08 80.85,23.19 81.17,25.83 v81.74,26.45 | HAND_MICRO2.61 117.64,41.01 111.81,35.18 98.12,35.18 90.98,28.04 90.98,26.11 v90.75,26.11
  Route2 0.254: 81.58,26.31 v81.74,26.45 83.16,27.89 89.28,27.89 v90.75,26.11
IDXPWM7  (via drill 0.38)
  Top 0.254: INDMID3.13 138.13,109.77 v139.57,108.33 | HAND_MICRO3.62 102.65,92.96 103.71,92.96 109.53,98.78 123.27,98.78 130.12,105.64 130.12,107.82 v130.71,108.41
  Route2 0.254: v130.71,108.41 139.52,108.38 v139.57,108.33
IDXPWM8  (via drill 0.38)
  Top 0.254: INDMID3.14 139.63,111.4 140.74,110.29 140.42,107.64 v139.85,107.02 | HAND_MICRO3.61 103.95,92.47 109.78,98.3 123.47,98.3 130.61,105.44 130.61,107.37 v130.84,107.37
  Route2 0.254: 140,107.16 v139.85,107.02 138.43,105.59 132.31,105.59 v130.84,107.37
LED0
  Top 0.254: HAND_MICRO.53 29.01,21.47 30.94,23.39 31.29,23.39 31.9,24 31.9,24.28 32.55,24.93 RED.1
LED1
  Top 0.254: GREEN.1 32.11,26.72 32.11,26.36 31.7,25.96 31.7,25.25 31.45,24.99 31.45,24.31 30.99,23.85 30.61,23.85 28.72,21.97 HAND_MICRO.54
LED2
  Top 0.254: HAND_MICRO.52 29.27,20.97 31.24,22.94 32.33,22.94 33.25,23.85 35.79,23.85 37.31,26.54 37.31,27.48 YELLOW.1
LED3
  Top 0.254: HAND_MICRO1.53 42.74,112.16 40.82,110.24 40.46,110.24 39.85,109.63 39.85,109.35 39.2,108.69 RED1.1
LED4
  Top 0.254: GREEN1.1 39.65,106.91 39.65,107.26 40.06,107.67 40.06,108.38 40.31,108.64 40.31,109.32 40.77,109.78 41.15,109.78 43.03,111.66 HAND_MICRO1.54
LED5
  Top 0.254: HAND_MICRO1.52 42.48,112.66 40.51,110.69 39.42,110.69 38.51,109.78 35.97,109.78 34.44,107.09 34.44,106.16 YELLOW1.1
LED6
  Top 0.254: HAND_MICRO2.53 117.6,45.01 115.67,43.08 115.32,43.08 114.71,42.47 114.71,42.19 114.05,41.54 RED2.1
LED7
  Top 0.254: GREEN2.1 114.5,39.75 114.5,40.11 114.91,40.51 114.91,41.22 115.16,41.48 115.16,42.16 115.62,42.62 116,42.62 117.89,44.51 HAND_MICRO2.54
LED8
  Top 0.254: HAND_MICRO2.52 117.34,45.51 115.37,43.54 114.28,43.54 113.36,42.62 110.82,42.62 109.3,39.93 109.3,39 YELLOW2.1
LED9
  Top 0.254: HAND_MICRO3.53 103.99,88.47 105.92,90.4 106.27,90.4 106.88,91.01 106.88,91.29 107.53,91.94 RED3.1
LED10
  Top 0.254: GREEN3.1 107.09,93.73 107.09,93.37 106.68,92.96 106.68,92.25 106.43,92 106.43,91.31 105.97,90.86 105.59,90.86 103.7,88.97 HAND_MICRO3.54
LED11
  Top 0.254: HAND_MICRO3.52 104.25,87.97 106.22,89.94 107.31,89.94 108.23,90.86 110.77,90.86 112.29,93.55 112.29,94.48 YELLOW3.1
MID1
  Top 0.381: INDMID.5 58.55,45.87
  Top 0.635: 58.55,45.87 57.33,46.05 56.67,46.97 55.02,47.93 52.93,50.01 47.4,50.01 MIDDLE.2
MID2
  Top 0.254: INDMID.3 60.53,46.99
  Top 0.381: 60.53,46.99 60.53,48.41
  Top 0.635: 60.53,48.41 60.17,48.62 59.31,49.1 55.55,49.1 53.57,51.08 MIDDLE.1
MID3
  Top 0.254: INDMID1.3 11.23,86.64
  Top 0.381: 11.23,86.64 11.23,85.22
  Top 0.635: 11.23,85.22 11.58,85.01 12.45,84.53 16.2,84.53 18.19,82.55 MIDDLE1.1
MID4
  Top 0.381: INDMID1.5 13.21,87.76
  Top 0.635: 13.21,87.76 14.43,87.58 15.09,86.67 16.74,85.7 18.82,83.62 24.36,83.62 MIDDLE1.2
MID5
  Top 0.254: INDMID2.3 86.08,19.48
  Top 0.381: 86.08,19.48 86.08,18.06
  Top 0.635: 86.08,18.06 86.44,17.86 87.3,17.37 91.06,17.37 93.04,15.39 MIDDLE2.1
MID6
  Top 0.381: INDMID2.5 88.06,20.6
  Top 0.635: 88.06,20.6 89.28,20.42 89.94,19.51 91.59,18.54 93.67,16.46 99.21,16.46 MIDDLE2.2
MID7
  Top 0.254: INDMID3.3 135.51,114
  Top 0.381: 135.51,114 135.51,115.42
  Top 0.635: 135.51,115.42 135.15,115.62 134.29,116.1 130.53,116.1 128.55,118.08 MIDDLE3.1
MID8
  Top 0.381: INDMID3.5 133.53,112.87
  Top 0.635: 133.53,112.87 132.31,113.06 131.65,113.97 130,114.94 127.91,117.02 122.38,117.02 MIDDLE3.2
MIDENC1  (via drill 0.38, 0.39)
  Top 0.254: v43.64,49.43 43.7,49.65 MIDDLE.5 | v31.22,26.62 30.86,26.62 29.21,24.97 HAND_MICRO.60
  Route2 0.254: v43.64,49.43 44.88,48.18 51.33,48.18 53.57,45.95 53.57,37.69 41.53,25.65 32.18,25.65 v31.22,26.62
MIDENC2  (via drill 0.38, 0.39)
  Top 0.254: MIDDLE.4 44.73,50.72 v44.73,49.58 | v30.96,25.65 30.63,25.65 29.45,24.47 HAND_MICRO.59
  Route2 0.254: v44.73,49.58 45.67,48.64 51.64,48.64 54.03,46.25 54.03,37.41 41.78,25.17 31.45,25.17 v30.96,25.65
MIDENC3  (via drill 0.38, 0.39)
  Top 0.254: MIDDLE1.4 27.03,82.91 v27.03,84.05 | v40.79,107.97 41.12,107.97 42.31,109.16 HAND_MICRO1.59
  Route2 0.254: v27.03,84.05 26.09,84.99 20.12,84.99 17.73,87.38 17.73,96.22 29.97,108.46 40.31,108.46 v40.79,107.97
MIDENC4  (via drill 0.38, 0.39)
  Top 0.254: v28.12,84.2 28.05,83.98 MIDDLE1.5 | v40.54,107.01 40.89,107.01 42.55,108.66 HAND_MICRO1.60
  Route2 0.254: v28.12,84.2 26.87,85.45 20.42,85.45 18.19,87.68 18.19,95.94 30.23,107.97 39.57,107.97 v40.54,107.01
MIDENC5  (via drill 0.38, 0.39)
  Top 0.254: MIDDLE2.4 101.88,15.75 v101.88,16.89 | v115.65,40.82 115.98,40.82 117.16,42.01 HAND_MICRO2.59
  Route2 0.254: v101.88,16.89 100.94,17.83 94.97,17.83 92.58,20.22 92.58,29.06 104.83,41.3 115.16,41.3 v115.65,40.82
MIDENC6  (via drill 0.38, 0.39)
  Top 0.254: v102.97,17.04 102.91,16.83 MIDDLE2.5 | v115.39,39.85 115.75,39.85 117.4,41.51 HAND_MICRO2.60
  Route2 0.254: v102.97,17.04 101.73,18.29 95.28,18.29 93.04,20.52 93.04,28.78 105.08,40.82 114.43,40.82 v115.39,39.85
MIDENC7  (via drill 0.38, 0.39)
  Top 0.254: MIDDLE3.4 119.71,117.72 v119.71,116.59 | v105.94,92.66 105.61,92.66 104.43,91.47 HAND_MICRO3.59
  Route2 0.254: v119.71,116.59 120.65,115.65 126.62,115.65 129.01,113.26 129.01,104.42 116.76,92.18 106.43,92.18 v105.94,92.66
MIDENC8  (via drill 0.38, 0.39)
  Top 0.254: v118.62,116.43 118.68,116.65 MIDDLE3.5 | v106.2,93.62 105.84,93.62 104.19,91.97 HAND_MICRO3.60
  Route2 0.254: v118.62,116.43 119.86,115.19 126.31,115.19 128.55,112.95 128.55,104.7 116.51,92.66 107.16,92.66 v106.2,93.62
MIDISEN  (via drill 0.38)
  Top 0.381: INDMID.4 59.7,47.47
  Top 0.635: 59.7,47.47 v58.8,47.7
  Bottom 0.635: v58.8,47.7 57.84,46.74 R7.2
MIDISEN1  (via drill 0.38)
  Top 0.381: INDMID1.4 12.05,86.16
  Top 0.635: 12.05,86.16 v12.95,85.93
  Bottom 0.635: v12.95,85.93 13.92,86.89 R23.2
MIDISEN2  (via drill 0.38)
  Top 0.381: INDMID2.4 86.91,19
  Top 0.635: 86.91,19 v87.81,18.77
  Bottom 0.635: v87.81,18.77 88.77,19.74 R39.2
MIDISEN3  (via drill 0.38)
  Top 0.381: INDMID3.4 134.68,114.48
  Top 0.635: 134.68,114.48 v133.78,114.71
  Bottom 0.635: v133.78,114.71 132.82,113.74 R55.2
MIDPWM1
  Top 0.254: 58.55,44.45 INDMID.7 56.91,44.39 54.18,41.66 54.18,39.04 47.88,32.74 34.04,32.74 28.26,26.97 HAND_MICRO.64
MIDPWM2
  Top 0.254: HAND_MICRO.63 28.5,26.47 34.29,32.26 48.08,32.26 54.66,38.84 54.66,41.43 56.98,43.74 INDMID.8
MIDPWM3
  Top 0.254: HAND_MICRO1.63 43.26,107.16 37.47,101.37 23.67,101.37 17.09,94.79 17.09,92.2 14.78,89.89 INDMID1.8
MIDPWM4
  Top 0.254: 13.21,89.18 INDMID1.7 14.84,89.24 17.58,91.97 17.58,94.59 23.88,100.89 37.72,100.89 43.49,106.66 HAND_MICRO1.64
MIDPWM5
  Top 0.254: HAND_MICRO2.63 118.11,40.01 112.32,34.21 98.53,34.21 91.95,27.64 91.95,25.04 89.63,22.73 INDMID2.8
MIDPWM6
  Top 0.254: 88.06,22.02 INDMID2.7 89.69,22.08 92.43,24.82 92.43,27.43 98.73,33.73 112.57,33.73 118.35,39.51 HAND_MICRO2.64
MIDPWM7
  Top 0.254: HAND_MICRO3.63 | HAND_MICRO3.63 103.48,93.47 109.27,99.26 123.06,99.26 129.64,105.84 129.64,108.43 131.96,110.75 INDMID3.8
MIDPWM8
  Top 0.254: 133.53,111.45 INDMID3.7 131.89,111.4 129.16,108.66 129.16,106.05 122.86,99.75 109.02,99.75 103.24,93.97 HAND_MICRO3.64
N$1  (via drill 0.38)
  Top 0.254: v34.49,26.44 35.86,26.44 RED.2
  Bottom 0.254: R14.1 34.02,25.97 v34.49,26.44
N$2  (via drill 0.38)
  Top 0.254: GREEN.2 33.98,28.67 v35,29.62
  Bottom 0.254: v35,29.62 34.81,29.64 R15.1
N$3  (via drill 0.38)
  Top 0.254: v37.64,29.72 36.41,28.82 YELLOW.2
  Bottom 0.254: R16.1 37.41,29.53 v37.64,29.72
N$4
  Top 0.254: INDMID.6 53.88,45.04 IMF.P$1
N$5
  Top 0.254: PKYRNG.6 27.05,37.72 25.86,36.52 PYF.P$1
N$6
  Top 0.254: THMB.6 28.35,15.04 TF.P$1
N$7
  Top 0.254: BOOTLOADER1.7 59.54,109.53 58.4,109.53 57.94,110.21 57.26,110.66 HAND_MICRO1.25
N$8
  Top 0.254: BOOTLOADER1.8 59.58,108.92 57.1,108.92 56.77,109.16 HAND_MICRO1.22
N$9  (via drill 0.38)
  Top 0.254: BOOTLOADER1.9 60.91,107.85 v59.84,107.85 | v57.25,109.75 56.61,110.16 HAND_MICRO1.24
  Bottom 0.254: v59.84,107.85 57.94,109.75 v57.25,109.75
N$10  (via drill 0.38)
  Top 0.254: BOOTLOADER1.13 64.17,108.92 v65.63,108.92 | v59.77,112.19 BOOTLOADER1.4 | v53.14,114.76 53.13,114.77 HAND_MICRO1.34
  Route15 0.254: v53.14,114.76 55.8,112.19 v59.77,112.19
  Bottom 0.254: v65.63,108.92 65.63,109.75 63.2,112.19 v59.77,112.19
N$11  (via drill 0.38)
  Top 0.254: HAND_MICRO1.15 53.13,103.24 | 53.13,103.24 53.13,101.31 C29.2 54.36,101.06 | C31.2 54.36,101.06 | 54.36,101.06 54.36,97.74 U$14.2 53.42,97.43 v52.68,97.41 | C30.2 50.7,101.06 50.39,100.76 v50.39,98.63 | HAND_MICRO1.16 53.63,103.74 53.13,103.24
  Bottom 0.254: v52.68,97.41 51.46,98.63 v50.39,98.63
N$12
  Top 0.381: INDMID1.9 12.31,91.64 13.23,91.64 15.12,93.53 C20.1
N$13
  Top 0.254: BOOTLOADER.7 12.22,24.11 13.36,24.11 13.82,23.42 14.5,22.97 HAND_MICRO.25
N$14
  Top 0.254: BOOTLOADER.8 12.18,24.71 14.66,24.71 14.98,24.47 HAND_MICRO.22
N$15  (via drill 0.38)
  Top 0.254: BOOTLOADER.9 10.85,25.78 v11.91,25.78 | v14.5,23.88 15.14,23.47 HAND_MICRO.24
  Bottom 0.254: v11.91,25.78 13.82,23.88 v14.5,23.88
N$16
  Top 0.381: C23.1 39.19,96.8 42.11,94.33 PKYRNG1.9
N$17  (via drill 0.38)
  Top 0.254: BOOTLOADER.13 7.58,24.71 v6.12,24.71 | v11.99,21.44 v11.98,21.44 BOOTLOADER.4 | v18.62,18.87 v18.63,18.86 HAND_MICRO.34
  Route15 0.254: v18.62,18.87 15.95,21.44 v11.99,21.44
  Bottom 0.254: v6.12,24.71 6.12,23.88 8.56,21.44 v11.99,21.44
N$18  (via drill 0.38)
  Top 0.254: HAND_MICRO.15 18.63,30.39 | 18.63,30.39 18.63,32.32 C10.2 17.4,32.57 | C12.2 17.4,32.57 | 17.4,32.57 17.4,35.89 U$3.2 18.34,36.2 v19.07,36.22 | C11.2 21.06,32.57 21.36,32.87 v21.36,35 | HAND_MICRO.16 18.13,29.89 18.63,30.39
  Bottom 0.254: v19.07,36.22 20.3,35 v21.36,35
N$19
  Top 0.381: C26.1 44.5,125.17 44.5,123.55 42.14,121.19 THMB1.9
N$20
  Top 0.381: THMB1.12 38.9,123.28 38.41,123.77 38.41,125.03 C27.1
N$21
  Top 0.381: INDMID.9 59.45,41.99 58.52,41.99 56.64,40.1 C1.1
N$22
  Top 0.381: C4.1 32.56,36.83 29.64,39.3 PKYRNG.9
N$23
  Top 0.381: C7.1 27.25,8.46 27.25,10.08 29.61,12.44 THMB.9
N$24
  Top 0.254: O16.3 15.41,14.5 | 18.01,17.48 18.08,17.47 HAND_MICRO.33
  Top 0.508: 15.41,14.5 16.56,14.5 18.01,15.92 18.01,17.48
N$25
  Top 0.381: THMB.12 32.85,10.35 33.35,9.86 33.35,8.59 C8.1
N$26
  Top 0.381: PKYRNG.12 30.36,42.19 31.55,43.84 31.82,44.05 32.38,44.91 33.86,44.91 C5.1
N$27
  Top 0.381: C2.1 63.03,41.26 INDMID.12
N$28
  Top 0.254: O16.1 13.89,16.63 | 16.48,19.3 HAND_MICRO.32
  Top 0.508: 13.89,16.63 13.89,17.25 15.98,19.3 16.48,19.3
N$29
  Top 0.381: PKYRNG1.12 41.39,91.44 40.21,89.79 39.93,89.58 39.37,88.72 37.9,88.72 C24.1
N$30
  Top 0.381: C21.1 8.72,92.36 INDMID1.12
N$31
  Top 0.254: RST.P$1 10.2,29.04 BOOTLOADER.10
N$32
  Top 0.254: R3.2 21.38,31.57 20.14,31.57 19.63,31.06 HAND_MICRO.13
N$33  (via drill 0.38)
  Top 0.254: 19.3,33.87 C11.1 20.45,33.94 20.45,35.31 21.06,35.92 21.74,35.92 22.38,35.28 R3.1 | 19.3,33.87 C10.1 | 19.3,33.87 19.3,31.8 19.13,31.62 HAND_MICRO.14 19.13,27.91 v18.95,27.58
  Bottom 0.254: v18.95,27.58 19.02,26.51 U$4.2
N$34  (via drill 0.38)
  Top 0.254: HAND_MICRO.17 14.64,26.97 v14.61,27 | v16.59,30.89 16.26,30.89 15.49,31.65 15.49,33.38 15.98,33.87 C12.1
  Bottom 0.254: v14.61,27 14.61,28.91 v16.59,30.89
N$35  (via drill 0.38)
  Top 0.254: USB.4 8.08,38.66 9.25,38.68 9.83,38.1 v9.83,33.53 | v17.61,24.25 17.41,24.25 17.14,23.98 HAND_MICRO.23 | BOOTLOADER.6 12.18,23.34 13.21,23.34 v13.74,22.43
  Bottom 0.254: v9.83,33.53 9.83,30.4 16.01,24.25 v17.61,24.25 16.27,22.44 v13.74,22.43
N$36
  Top 0.254: O1.3 56.34,119.13 | 53.75,116.15 53.68,116.16 HAND_MICRO1.33
  Top 0.508: 56.34,119.13 55.19,119.13 53.75,117.71 53.75,116.15
N$37
  Top 0.254: O1.1 57.86,117 | 55.27,114.33 HAND_MICRO1.32
  Top 0.508: 57.86,117 57.86,116.38 55.78,114.33 55.27,114.33
N$38
  Top 0.254: RST1.P$1 61.55,104.59 BOOTLOADER1.10
N$39
  Top 0.254: R19.2 50.37,102.06 51.61,102.06 52.13,102.57 HAND_MICRO1.13
N$40  (via drill 0.38)
  Top 0.254: 52.45,99.76 C30.1 51.31,99.69 51.31,98.32 50.7,97.71 50.01,97.71 49.38,98.35 R19.1 | 52.45,99.76 C29.1 | 52.45,99.76 52.45,101.83 52.63,102 HAND_MICRO1.14 52.63,105.72 v52.81,106.05
  Bottom 0.254: v52.81,106.05 52.73,107.12 U$15.2
N$41  (via drill 0.38)
  Top 0.254: HAND_MICRO1.17 57.12,106.66 v57.15,106.63 | v55.17,102.74 55.5,102.74 56.26,101.98 56.26,100.25 55.77,99.76 C31.1
  Bottom 0.254: v57.15,106.63 57.15,104.72 v55.17,102.74
N$42  (via drill 0.38)
  Top 0.254: USB1.4 63.68,94.97 62.51,94.94 61.92,95.53 v61.92,100.1 | v54.14,109.38 54.34,109.38 54.61,109.65 HAND_MICRO1.23 | BOOTLOADER1.6 59.57,110.29 58.55,110.29 v58.01,111.2
  Bottom 0.254: v61.92,100.1 61.92,103.23 55.74,109.38 v54.14,109.38 55.48,111.19 v58.01,111.2
N$43  (via drill 0.38)
  Top 0.254: v37.26,107.19 35.9,107.19 RED1.2
  Bottom 0.254: R30.1 37.73,107.66 v37.26,107.19
N$44  (via drill 0.38)
  Top 0.254: GREEN1.2 37.78,104.96 v36.75,104.01
  Bottom 0.254: v36.75,104.01 36.94,103.99 R31.1
N$45  (via drill 0.38)
  Top 0.254: v34.11,103.91 35.34,104.81 YELLOW1.2
  Bottom 0.254: R32.1 34.34,104.1 v34.11,103.91
N$46
  Top 0.254: INDMID1.6 17.87,88.59 IMF1.P$1
N$47
  Top 0.254: PKYRNG1.6 44.7,95.91 45.9,97.1 PYF1.P$1
N$48
  Top 0.254: THMB1.6 43.4,118.59 TF1.P$1
N$49
  Top 0.254: BOOTLOADER2.7 134.39,42.37 133.25,42.37 132.79,43.05 132.11,43.51 HAND_MICRO2.25
N$50
  Top 0.254: BOOTLOADER2.8 134.43,41.76 131.95,41.76 131.63,42.01 HAND_MICRO2.22
N$51  (via drill 0.38)
  Top 0.254: BOOTLOADER2.9 135.76,40.69 v134.7,40.69 | v132.1,42.6 131.47,43.01 HAND_MICRO2.24
  Bottom 0.254: v134.7,40.69 132.79,42.6 v132.1,42.6
N$52  (via drill 0.38)
  Top 0.254: BOOTLOADER2.13 139.03,41.76 v140.49,41.76 | v134.62,45.03 BOOTLOADER2.4 | v127.99,47.6 v127.98,47.61 HAND_MICRO2.34
  Route15 0.254: v127.99,47.6 130.66,45.03 v134.62,45.03
  Bottom 0.254: v140.49,41.76 140.49,42.6 138.05,45.03 v134.62,45.03
N$53  (via drill 0.38)
  Top 0.254: HAND_MICRO2.15 127.98,36.08 | 127.98,36.08 127.98,34.16 C48.2 129.21,33.91 | C50.2 129.21,33.91 | 129.21,33.91 129.21,30.59 U$26.2 128.27,30.28 v127.53,30.25 | C49.2 125.55,33.91 125.25,33.6 v125.25,31.47 | HAND_MICRO2.16 128.48,36.58 127.98,36.08
  Bottom 0.254: v127.53,30.25 126.31,31.47 v125.25,31.47
N$54
  Top 0.381: INDMID2.9 87.16,24.49 88.09,24.49 89.97,26.37 C39.1
N$55
  Top 0.381: C42.1 114.05,29.64 116.97,27.17 PKYRNG2.9
N$56
  Top 0.381: C45.1 119.36,58.01 119.36,56.39 117,54.03 THMB2.9
N$57
  Top 0.381: THMB2.12 113.76,56.12 113.26,56.62 113.26,57.88 C46.1
N$58
  Top 0.381: PKYRNG2.12 116.25,24.28 115.06,22.63 114.78,22.42 114.22,21.57 112.75,21.57 C43.1
N$59
  Top 0.381: C40.1 83.58,25.21 INDMID2.12
N$60
  Top 0.254: O2.3 131.2,51.97 | 128.6,49 128.53,49.01 HAND_MICRO2.33
  Top 0.508: 131.2,51.97 130.05,51.97 128.6,50.55 128.6,49
N$61
  Top 0.254: O2.1 132.72,49.84 | 130.12,47.17 HAND_MICRO2.32
  Top 0.508: 132.72,49.84 132.72,49.23 130.63,47.17 130.12,47.17
N$62
  Top 0.254: RST2.P$1 136.41,37.43 BOOTLOADER2.10
N$63
  Top 0.254: R35.2 125.22,34.9 126.47,34.9 126.98,35.41 HAND_MICRO2.13
N$64  (via drill 0.38)
  Top 0.254: 127.31,32.6 C49.1 126.16,32.54 126.16,31.17 125.55,30.56 124.87,30.56 124.23,31.19 R35.1 | 127.31,32.6 C48.1 | 127.31,32.6 127.31,34.67 127.48,34.85 HAND_MICRO2.14 127.48,38.56 v127.66,38.89
  Bottom 0.254: v127.66,38.89 127.58,39.96 U$27.2
N$65  (via drill 0.38)
  Top 0.254: HAND_MICRO2.17 131.97,39.51 v132,39.47 | v130.02,35.59 130.35,35.59 131.12,34.82 131.12,33.1 130.62,32.6 C50.1
  Bottom 0.254: v132,39.47 132,37.57 v130.02,35.59
N$66  (via drill 0.38)
  Top 0.254: USB2.4 138.53,27.81 137.36,27.79 136.78,28.37 v136.78,32.94 | v129,42.23 129.2,42.23 129.46,42.49 HAND_MICRO2.23 | BOOTLOADER2.6 134.43,43.13 133.4,43.13 v132.87,44.04
  Bottom 0.254: v136.78,32.94 136.78,36.07 130.6,42.23 v129,42.23 130.34,44.03 v132.87,44.04
N$67  (via drill 0.38)
  Top 0.254: v112.12,40.03 110.75,40.03 RED2.2
  Bottom 0.254: R46.1 112.58,40.5 v112.12,40.03
N$68  (via drill 0.38)
  Top 0.254: GREEN2.2 112.63,37.8 v111.61,36.85
  Bottom 0.254: v111.61,36.85 111.8,36.83 R47.1
N$69  (via drill 0.38)
  Top 0.254: v108.97,36.75 110.19,37.65 YELLOW2.2
  Bottom 0.254: R48.1 109.19,36.95 v108.97,36.75
N$70
  Top 0.254: INDMID2.6 92.73,21.43 IMF2.P$1
N$71
  Top 0.254: PKYRNG2.6 119.56,28.75 120.75,29.95 PYF2.P$1
N$72
  Top 0.254: THMB2.6 118.26,51.43 TF2.P$1
N$73
  Top 0.254: BOOTLOADER3.7 87.2,91.11 88.34,91.11 88.8,90.42 89.48,89.97 HAND_MICRO3.25
N$74
  Top 0.254: BOOTLOADER3.8 87.16,91.72 89.64,91.72 89.96,91.47 HAND_MICRO3.22
N$75  (via drill 0.38)
  Top 0.254: BOOTLOADER3.9 85.83,92.79 v86.89,92.79 | v89.48,90.88 90.12,90.47 HAND_MICRO3.24
  Bottom 0.254: v86.89,92.79 88.8,90.88 v89.48,90.88
N$76  (via drill 0.38)
  Top 0.254: BOOTLOADER3.13 82.56,91.72 v81.1,91.72 | v86.97,88.44 v86.97,88.45 BOOTLOADER3.4 | v93.6,85.88 93.61,85.87 HAND_MICRO3.34
  Route15 0.254: v93.6,85.88 90.93,88.44 v86.97,88.44
  Bottom 0.254: v81.1,91.72 81.1,90.88 83.54,88.44 v86.97,88.44
N$77  (via drill 0.38)
  Top 0.254: HAND_MICRO3.15 93.61,97.4 | 93.61,97.4 93.61,99.32 C67.2 92.38,99.57 | C69.2 92.38,99.57 | 92.38,99.57 92.38,102.89 U$38.2 93.32,103.2 v94.06,103.23 | C68.2 96.04,99.57 96.34,99.87 v96.34,102.01 | HAND_MICRO3.16 93.11,96.9 93.61,97.4
  Bottom 0.254: v94.06,103.23 95.28,102.01 v96.34,102.01
N$78
  Top 0.381: INDMID3.9 134.43,108.99 133.5,108.99 131.62,107.11 C58.1
N$79
  Top 0.381: C61.1 107.54,103.83 104.62,106.31 PKYRNG3.9
N$80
